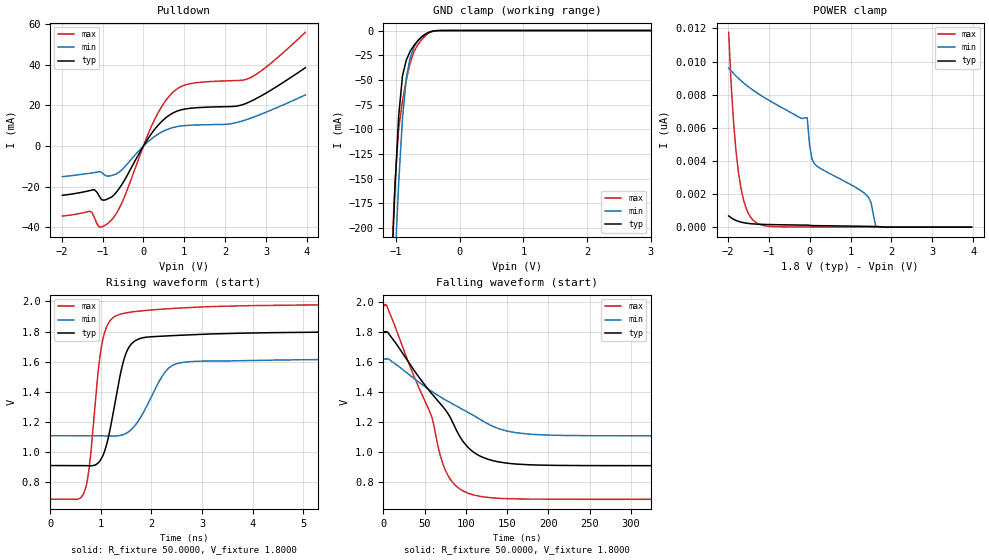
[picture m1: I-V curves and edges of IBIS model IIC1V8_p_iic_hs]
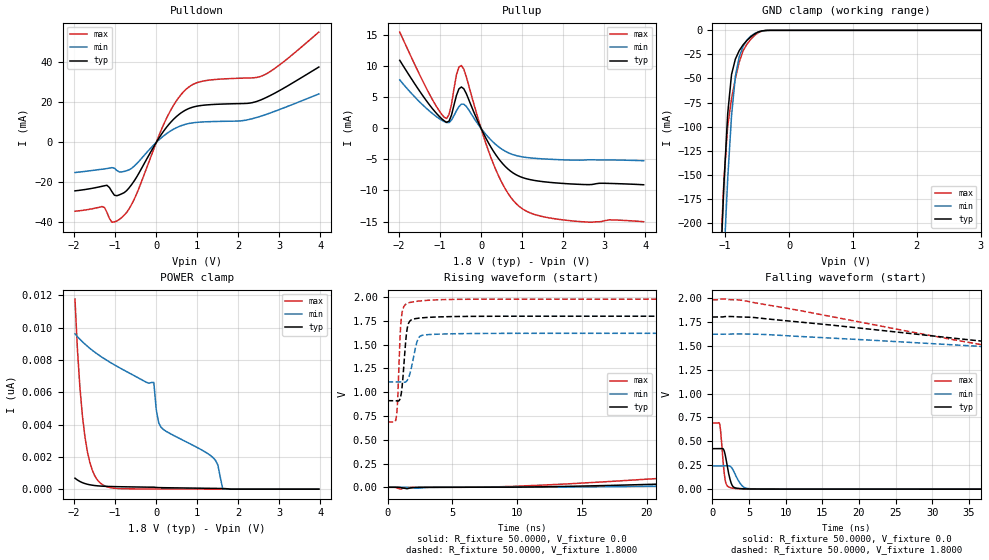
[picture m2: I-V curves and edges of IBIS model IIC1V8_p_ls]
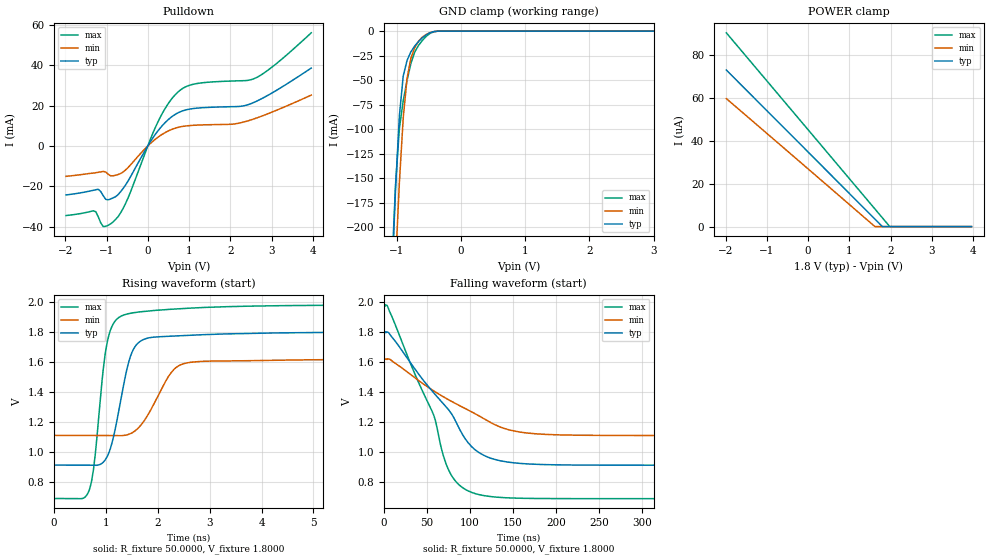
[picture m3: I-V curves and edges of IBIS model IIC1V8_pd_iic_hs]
| IBIS file qfn48_1p8v.ibs generated by Viper version: 2020.12.17
[IBIS Ver]   5.0
[Comment Char]   |_char
[File Name]   qfn48_1p8v.ibs
[File Rev]   1.3
[Date]   Thu Dec 17 17:48:23 2020
[Source]   NXP Viper 2020.12.17
[Notes]
[Disclaimer] IMPORTANT NOTICE
  This information is provided on an AS IS basis and without warranty.
  IN NO EVENT SHALL NXP BE LIABLE FOR INCIDENTAL OR CONSEQUENTIAL
  DAMAGES ARISING FROM USE OF THIS INFORMATION. THIS DISCLAIMER OF
  WARRANTY EXTENDS TO THE USER OF THE INFORMATION, AND TO THEIR CUSTOMERS
  OR USERS OF PRODUCTS  AND IS IN LIEU OF ALL WARRANTIES WHETHER EXPRESS,
  IMPLIED, OR STATUTORY, INCLUDING IMPLIED WARRANTIES OF MERCHANTABILITY
  OR FITNESS FOR PARTICULAR PURPOSE.
  NXP does not represent or warrant that the information furnished
  hereunder is free of infringement of any third party patents,
  copyrights, trade secrets, or other intellectual property rights.
  NXP does not represent or warrant that the information is free of
  defect, or that it meets any particular standard, requirements or need
  of the user of the infomation or their customers.
  NXP reserves the right to change the information in this file
  without notice.
   http://www.nxp.com
[Copyright]   (C) Copyright NXP 2004 - 2020, All Rights Reserved.
|   qfn48
[Component]   qfn48
[Manufacturer]   NXP
[Package]
| variable   typ   min   max
R_pkg   0.17546   0.085233   0.21913
L_pkg   1.979e-9   1.305e-9   2.456e-9
C_pkg   2.005e-13   1.705e-13   3.136e-13
[Pin] signal_name   model_name   R_pin   L_pin   C_pin
1   OPAMP2_INN   NC   0.19686   2.31e-9   1.975e-13
2   P0_1   gpio   0.19885   2.125e-9  1.995e-13
3   P1_0   gpio   0.18462   1.924e-9  1.916e-13
4   P0_11   gpio   0.16868   1.868e-9  1.705e-13
5   VDDIO_1   POWER   NA   NA   NA
6   VDDA   POWER   NA   NA   NA
7   VREF_OUT   NC   0.085233  1.305e-9  2.26e-13
8   VREFP   NC   0.088717  1.309e-9  2.417e-13
9   VREFN   GND   NA   NA   NA
10   P0_16   gpio   0.17435   1.987e-9  1.764e-13
11   P0_10   gpio   0.18496   2.194e-9  1.962e-13
12   P0_15   gpio   0.20527   2.456e-9  2.081e-13
13   P0_8   gpio   0.19119   2.293e-9  1.955e-13
14   OPAMP0_INN   NC   0.1741   2.073e-9  2.101e-13
15   P0_27   gpio   0.16311   1.909e-9  1.814e-13
16   OPAMP1_INN   NC   0.16129   1.801e-9  1.909e-13
17   RESETN   gpio   0.16527   1.717e-9  1.895e-13
18   VDD_CORE   POWER   NA   NA   NA
19   P0_17   gpio   0.16074   1.801e-9  1.861e-13
20   P0_7   gpio   0.1631   1.762e-9  1.925e-13
21   VDDIO_1   POWER   NA   NA   NA
22   VSS_MAIN   GND   NA   NA   NA
23   LX   NC   0.10755   1.361e-9  3.136e-13
24   VDD_MAIN_PWR   NC   NA   NA   NA
25   VBAT   NC   0.21039   2.199e-9  2.126e-13
26   P0_0   gpio   0.19752   2.015e-9  2.122e-13
27   P0_9   gpio   0.17432   1.951e-9  1.886e-13
28   P0_18   gpio   0.16396   1.852e-9  1.719e-13
29   P1_1   gpio   0.1654   1.786e-9  1.75e-13
30   P0_26   gpio   0.16144   1.856e-9  1.764e-13
31   P1_2   gpio   0.16991   1.948e-9  1.848e-13
32   P1_3   gpio   0.18887   2.054e-9  1.928e-13
33   P0_24   gpio   0.17001   1.885e-9  1.791e-13
34   P0_13   iic   0.18016   2.084e-9  1.944e-13
35   P0_14   iic   0.19867   2.298e-9  2.017e-13
36   P0_20   gpio   0.21913   2.324e-9  2.127e-13
37   P0_21   gpio   0.20869   2.216e-9  2.193e-13
38   P0_2   gpio   0.21473   2.265e-9  2.308e-13
39   P0_19   gpio   0.18997   2.14e-9   2.172e-13
40   P0_3   gpio   0.17488   1.926e-9  2.022e-13
41   VDDIO_2   POWER   NA   NA   NA
42   P0_4   gpio   0.16342   1.796e-9  1.814e-13
43   P0_6   gpio   0.16772   1.736e-9  1.992e-13
44   P0_5   gpio   0.16504   1.891e-9  1.879e-13
45   P0_29   gpio   0.16929   1.996e-9  1.98e-13
46   P1_11   gpio   0.18558   2.171e-9  1.964e-13
47   P0_30   gpio   0.20664   2.318e-9  2.205e-13
48   P2_1   gpio   0.1989   2.278e-9  1.972e-13
49   VSS   GND   NA   NA   NA
[Pin Mapping]   pulldown_ref   pullup_ref
1   NC   NC
2   VSS   VDDA
3   VSS   VDDA
4   VSS   VDDA
5   NC   VDDIO_1
6   NC   VDDA
7   NC   NC
8   NC   NC
9   VREFN   NC
10   VSS   VDDA
11   VSS   VDDA
12   VSS   VDDA
13   VSS   VDDA
14   NC   NC
15   VSS   VDDA
16   NC   NC
17   VSS   VDDIO_1
18   NC   VDD_CORE
19   VSS   VDDIO_1
20   VSS   VDDIO_1
21   NC   VDDIO_1
22   VSS_MAIN   NC
23   NC   NC
24   NC   NC
25   NC   NC
26   VSS   VDDIO_2
27   VSS   VDDIO_2
28   VSS   VDDIO_2
29   VSS   VDDIO_2
30   VSS   VDDIO_2
31   VSS   VDDIO_2
32   VSS   VDDIO_2
33   VSS   VDDIO_2
34   VSS   VDDIO_2
35   VSS   VDDIO_2
36   VSS   VDDIO_2
37   VSS   VDDIO_2
38   VSS   VDDIO_2
39   VSS   VDDIO_2
40   VSS   VDDIO_2
41   NC   VDDIO_2
42   VSS   VDDIO_2
43   VSS   VDDIO_2
44   VSS   VDDIO_2
45   VSS   VDDIO_2
46   VSS   VDDIO_2
47   VSS   VDDIO_2
48   VSS   VDDA
49   VSS   NC
|*   Model Selector   *
[Model Selector] gpio
MFIO1V8_pd_hs   EPUN=1 EPD=1 EHS=1
MFIO1V8_pd_ls   EPUN=1 EPD=1 EHS=0
MFIO1V8_pu_hs   EPUN=0 EPD=0 EHS=1
MFIO1V8_pu_ls   EPUN=0 EPD=0 EHS=0
MFIO1V8_p_hs   EPUN=1 EPD=0 EHS=1
MFIO1V8_p_ls   EPUN=1 EPD=0 EHS=0
MFIO1V8_r_hs   EPUN=0 EPD=1 EHS=1
MFIO1V8_r_ls   EPUN=0 EPD=1 EHS=0
[Model Selector] iic
IIC1V8_pd_hs   EGP=1 EPUN=1 EPD=1 EHS=1
IIC1V8_pd_ls   EGP=1 EPUN=1 EPD=1 EHS=0
IIC1V8_p_hs   EGP=1 EPUN=1 EPD=0 EHS=1
IIC1V8_p_ls   EGP=1 EPUN=1 EPD=0 EHS=0
IIC1V8_pu_hs   EGP=1 EPUN=0 EPD=0 EHS=1
IIC1V8_pu_ls   EGP=1 EPUN=0 EPD=0 EHS=0
IIC1V8_r_hs   EGP=1 EPUN=0 EPD=1 EHS=1
IIC1V8_r_ls   EGP=1 EPUN=0 EPD=1 EHS=0
IIC1V8_pd_iic_hs   EGP=0 ECS=0 EPUN=1 EPD=1
IIC1V8_p_iic_hs   EGP=0 ECS=0 EPUN=1 EPD=0
IIC1V8_pu_iic_hs   EGP=0 ECS=0 EPUN=0 EPD=0
IIC1V8_r_iic_hs   EGP=0 ECS=0 EPUN=0 EPD=1
IIC1V8_pd_iic_pu_hs   EGP=0 ECS=1 EPUN=1 EPD=1 SSEL=1
IIC1V8_p_iic_pu_hs   EGP=0 ECS=1 EPUN=1 EPD=0 SSEL=1
IIC1V8_pu_iic_pu_hs   EGP=0 ECS=1 EPUN=0 EPD=0 SSEL=1
IIC1V8_r_iic_pu_hs   EGP=0 ECS=1 EPUN=0 EPD=1 SSEL=1
| End [Component] qfn48
| Models and submodels in the file (24): IIC1V8_p_hs (I/O), IIC1V8_p_iic_hs (I/O_open_drain), IIC1V8_p_iic_pu_hs (I/O_open_drain), IIC1V8_p_ls (I/O), IIC1V8_pd_hs (I/O), IIC1V8_pd_iic_hs (I/O_open_drain), IIC1V8_pd_iic_pu_hs (I/O_open_drain), IIC1V8_pd_ls (I/O), IIC1V8_pu_hs (I/O), IIC1V8_pu_iic_hs (I/O_open_drain), IIC1V8_pu_iic_pu_hs (I/O_open_drain), IIC1V8_pu_ls (I/O), IIC1V8_r_hs (I/O), IIC1V8_r_iic_hs (I/O_open_drain), IIC1V8_r_iic_pu_hs (I/O_open_drain), IIC1V8_r_ls (I/O), MFIO1V8_p_hs (I/O), MFIO1V8_p_ls (I/O), MFIO1V8_pd_hs (I/O), MFIO1V8_pd_ls (I/O), MFIO1V8_pu_hs (I/O), MFIO1V8_pu_ls (I/O), MFIO1V8_r_hs (I/O), MFIO1V8_r_ls (I/O)
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[Model] IIC1V8_p_iic_hs
|   Model IIC1V8_p_iic_hs
| This model was characterised for following simulation conditions:
| External (pad) voltage:
|   - Typ: 1.8V,   - Min: 1.62V,   - Max: 1.98V
| Library cells for typ/min/max conditions are connected as defined below:
|  IO - External Pad
|  A - Core Input
|  EN - Output Buffer Enable
|  BOOST - vdde
|  ECS - gnd
|  EGP - gnd
|  ENZI - vdd
|  EPD - gnd
|  EPUN - vdd
|  ZI - NC
|  ZIF - NC
|  gnd - gnd
|  gnde - gnde
|  vdd - vdd
|  vdde - vdde
| All other pins connected to ground
Model_type I/O_open_drain
Polarity   Non-Inverting
Enable   Active-Low
Vinl =   0.5400V
Vinh =   1.2600V
Vmeas =  0.9000V
Cref =   0.0F
Rref =   1000.000
Vref =   1.8000V
C_comp   3.6454pF   3.5038pF   3.7808pF
|C_comp_pullup   0.9524pF   0.9269pF   0.9624pF
|C_comp_pulldown   2.3410pF   2.4924pF   2.1971pF
[Model Spec]
| variable   typ   min   max
Vinh   0.5400V   0.4860V   0.5940V
Vinl   1.2600V   1.1340V   1.3860V
Vmeas   0.9000V   0.8100V   0.9900V
Vref   1.8000V   1.6200V   1.9800V
Cref   0.0F   0.0F   0.0F
Rref   1.0000k   1.0000k   1.0000k
[Temperature Range]   25.0000   0.1250k   -40.0000
[Voltage Range]   1.8000V   1.6200V   1.9800V
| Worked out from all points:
|   slope of the pulldown table from 0 to 0.27 V, typ, clamps not added: 33.4 ohm
|   GND clamp passes 1 mA (typ) near -0.44 V on its own axis
|   rising waveform, R_fixture 50.0000, V_fixture 1.8000: 20-80 % time 321ps typ, 491ps min, 237ps max; typ from 0.911 V to 1.8 V
|   falling waveform, R_fixture 50.0000, V_fixture 1.8000: 20-80 % time 66.9ns typ, 88.7ns min, 48.9ns max; typ from 1.8 V to 0.911 V
[Pulldown]
|Voltage   I(typ)   I(min)   I(max)
-1.98V    -24.22mA   -15.04mA   -34.42mA
-1.32V    -21.94mA   -13.4mA    -32.06mA
-1.2V     -21.45mA   -13.05mA   -35.06mA
-1.08V    -24.63mA   -12.6mA    -39.9mA
-900mV    -26.23mA   -14.78mA   -38.53mA
-540mV    -19.33mA   -11.9mA    -28.53mA
300mV     8.856mA    5.096mA    14.12mA
720mV     16.26mA    9.117mA    26.48mA
1.14V     18.6mA     10.26mA    30.69mA
2.1V      19.45mA    10.9mA     32.16mA
2.58V     21.61mA    13.44mA    33.34mA
3.96V     38.56mA    25.19mA    55.99mA
[GND_clamp]
|Voltage   I(typ)   I(min)   I(max)
-1.98V    -2.104A    -2.075A    -2.136A
-1.08V    -259.3mA   -333mA     -246.9mA
-1.02V    -161.8mA   -238.7mA   -157.1mA
-960mV    -86.74mA   -154.7mA   -99.46mA
-900mV    -45.95mA   -88.82mA   -71.05mA
-840mV    -29.9mA    -47.99mA   -50.25mA
-780mV    -21.15mA   -27.64mA   -32.98mA
-720mV    -15.16mA   -16.87mA   -21.26mA
-660mV    -10.56mA   -10.24mA   -14.56mA
-540mV    -3.788mA   -3.398mA   -5.292mA
-300mV    -15.94uA   -36uA      -16.34uA
3.96V     0A         0A         0A
[POWER_clamp]
|Voltage   I(typ)   I(min)   I(max)
-1.98V    679.6pA    9.61nA     11.76nA
-1.86V    475.2pA    9.277nA    6.313nA
-1.74V    349.2pA    8.982nA    3.292nA
-1.56V    245.6pA    8.597nA    1.186nA
-1.32V    186pA      8.161nA    293.2pA
-60mV     124.8pA    6.606nA    14.31pA
0V        105.5pA    4.916nA    11.81pA
120mV     93.21pA    3.82nA     10.91pA
1.38V     50pA       1.96nA     2.877pA
1.5V      45.28pA    1.501nA    2.149pA
1.62V     39.18pA    0A         1.42pA
3.96V     0A         0A         0A
[Ramp]
| variable   typ   min   max
dV/dt_r  0.5334/0.3209n   0.3066/0.4909n   0.7753/0.2369n
dV/dt_f  0.5334/66.9323n   0.3066/88.7325n   0.7753/48.9497n
R_load = 50.0000
[Rising Waveform]
R_fixture= 50.0000
V_fixture= 1.8000
V_fixture_min= 1.6200
V_fixture_max= 1.9800
|time   V(typ)   V(min)   V(max)
0s        911mV      1.109V     687.8mV
683.3ps   910.2mV    1.109V     745.5mV
780.5ps   909.1mV    1.109V     927.7mV
1.017ns   961.1mV    1.108V     1.71V
1.277ns   1.32V      1.107V     1.9V
1.506ns   1.663V     1.126V     1.925V
1.797ns   1.757V     1.237V     1.938V
2.547ns   1.776V     1.591V     1.956V
6.124ns   1.798V     1.616V     1.979V
1us       1.8V       1.62V      1.98V
[Falling Waveform]
R_fixture= 50.0000
V_fixture= 1.8000
V_fixture_min= 1.6200
V_fixture_max= 1.9800
|time   V(typ)   V(min)   V(max)
0s        1.8V       1.62V      1.98V
4.033ns   1.8V       1.621V     1.975V
57.1ns    1.4V       1.41V      1.258V
68.97ns   1.323V     1.369V     978.6mV
76.93ns   1.269V     1.343V     860.5mV
95.01ns   1.085V     1.288V     749mV
110.3ns   997.3mV    1.242V     715.6mV
148.2ns   929.5mV    1.144V     692.6mV
208ns     913.4mV    1.113V     688.4mV
1us       911.1mV    1.109V     687.9mV
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[Model] IIC1V8_p_ls
|   Model IIC1V8_p_ls
| This model was characterised for following simulation conditions:
| External (pad) voltage:
|   - Typ: 1.8V,   - Min: 1.62V,   - Max: 1.98V
| Library cells for typ/min/max conditions are connected as defined below:
|  IO - External Pad
|  A - Core Input
|  EN - Output Buffer Enable
|  BOOST - vdde
|  EGP - vdd
|  EHS - gnd
|  ENZI - vdd
|  EPD - gnd
|  EPUN - vdd
|  ZI - NC
|  ZIF - NC
|  gnd - gnd
|  gnde - gnde
|  vdd - vdd
|  vdde - vdde
| All other pins connected to ground
Model_type I/O
Polarity   Non-Inverting
Enable   Active-Low
Vinl =   0.5400V
Vinh =   1.2600V
Vmeas =  0.9000V
Cref =   0.0F
Rref =   1.0000k
Vref =   0.0V
C_comp   3.6452pF   3.5037pF   3.7805pF
|C_comp_pullup   0.9521pF   0.9262pF   0.9623pF
|C_comp_pulldown   2.3411pF   2.4927pF   2.1971pF
[Model Spec]
| variable   typ   min   max
Vinh   0.5400V   0.4860V   0.5940V
Vinl   1.2600V   1.1340V   1.3860V
Vmeas   0.9000V   0.8100V   0.9900V
[Temperature Range]   25.0000   0.1250k   -40.0000
[Voltage Range]   1.8000V   1.6200V   1.9800V
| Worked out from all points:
|   slope of the pulldown table from 0 to 0.27 V, typ, clamps not added: 33.4 ohm
|   slope of the pullup table from 0 to 0.27 V, typ, clamps not added: 80.7 ohm
|   GND clamp passes 1 mA (typ) near -0.44 V on its own axis
|   rising waveform, R_fixture 50.0000, V_fixture 0.0: 20-80 % time 70.1ns typ, 82ns min, 57.1ns max; typ from 0 V to 0.423 V
|   rising waveform, R_fixture 50.0000, V_fixture 1.8000: 20-80 % time 319ps typ, 487ps min, 235ps max; typ from 0.911 V to 1.8 V
|   falling waveform, R_fixture 50.0000, V_fixture 0.0: 20-80 % time 672ps typ, 1.04ns min, 474ps max; typ from 0.423 V to 0 V
|   falling waveform, R_fixture 50.0000, V_fixture 1.8000: 20-80 % time 66.9ns typ, 88.7ns min, 49ns max; typ from 1.8 V to 0.911 V
[Pulldown]
|Voltage   I(typ)   I(min)   I(max)
-1.98V    -24.22mA   -15.04mA   -34.42mA
-1.32V    -21.94mA   -13.4mA    -32.06mA
-1.2V     -21.45mA   -13.05mA   -35.06mA
-1.08V    -24.63mA   -12.6mA    -39.9mA
-900mV    -26.23mA   -14.78mA   -38.53mA
-720mV    -24.07mA   -14.13mA   -34.99mA
-540mV    -19.33mA   -11.9mA    -28.53mA
300mV     8.856mA    5.096mA    14.12mA
720mV     16.26mA    9.117mA    26.48mA
1.14V     18.6mA     10.26mA    30.69mA
2.58V     21.56mA    13.35mA    33.32mA
3.96V     37.73mA    24.28mA    55.2mA
[Pullup]
|Voltage   I(typ)   I(min)   I(max)
-1.98V    10.95mA    7.799mA    15.5mA
-1.32V    4.346mA    3.159mA    6.304mA
-900mV    1.218mA    1.094mA    1.804mA
-780mV    1.156mA    929.2uA    2.224mA
-600mV    5.286mA    2.831mA    8.611mA
-480mV    6.667mA    3.906mA    10.12mA
-420mV    6.372mA    3.889mA    9.539mA
360mV     -4.265mA   -2.608mA   -6.666mA
660mV     -6.57mA    -3.917mA   -10.5mA
960mV     -7.8mA     -4.537mA   -12.74mA
2.04V     -8.889mA   -5.075mA   -14.77mA
3.96V     -9.081mA   -5.209mA   -15.04mA
[GND_clamp]
|Voltage   I(typ)   I(min)   I(max)
-1.98V    -2.104A    -2.075A    -2.136A
-1.08V    -259.3mA   -333mA     -246.9mA
-1.02V    -161.8mA   -238.7mA   -157.1mA
-960mV    -86.74mA   -154.7mA   -99.46mA
-900mV    -45.95mA   -88.82mA   -71.05mA
-840mV    -29.9mA    -47.99mA   -50.25mA
-780mV    -21.15mA   -27.64mA   -32.98mA
-720mV    -15.16mA   -16.87mA   -21.26mA
-660mV    -10.56mA   -10.24mA   -14.56mA
-540mV    -3.788mA   -3.398mA   -5.292mA
-300mV    -15.94uA   -36uA      -16.34uA
3.96V     0A         0A         0A
[POWER_clamp]
|Voltage   I(typ)   I(min)   I(max)
-1.98V    679.6pA    9.61nA     11.76nA
-1.86V    475.2pA    9.277nA    6.313nA
-1.74V    349.2pA    8.982nA    3.292nA
-1.56V    245.6pA    8.597nA    1.186nA
-1.32V    186pA      8.161nA    293.2pA
-60mV     124.8pA    6.606nA    14.31pA
0V        105.5pA    4.916nA    11.81pA
120mV     93.21pA    3.82nA     10.91pA
1.38V     50pA       1.96nA     2.877pA
1.5V      45.28pA    1.501nA    2.149pA
1.62V     39.18pA    0A         1.42pA
3.96V     0A         0A         0A
[Ramp]
| variable   typ   min   max
dV/dt_r  0.2539/70.1178n   0.1457/81.9302n   0.4150/57.0489n
dV/dt_f  0.5334/66.9358n   0.3066/88.6649n   0.7753/48.9538n
R_load = 50.0000
[Rising Waveform]
R_fixture= 50.0000
V_fixture= 0.0
V_fixture_min= 0.0
V_fixture_max= 0.0
|time   V(typ)   V(min)   V(max)
0s        602.8pV    52.95nV    41.9pV
1.012ns   -3.31mV    192.5uV    -19.98mV
1.632ns   -11.39mV   -2.738mV   -1.795mV
12.68ns   6.299mV    1.388mV    27.19mV
45.88ns   145.4mV    64.89mV    304.8mV
84.55ns   285.2mV    143.4mV    561.1mV
103.3ns   339.8mV    172mV      629.2mV
134ns     392.1mV    207.9mV    672.5mV
250.9ns   422.4mV    241.3mV    691.3mV
1us       423.2mV    242.8mV    691.7mV
[Rising Waveform]
R_fixture= 50.0000
V_fixture= 1.8000
V_fixture_min= 1.6200
V_fixture_max= 1.9800
|time   V(typ)   V(min)   V(max)
0s        911mV      1.109V     687.8mV
685.2ps   909.5mV    1.109V     745.1mV
787ps     907.1mV    1.109V     945.8mV
1.007ns   951.3mV    1.108V     1.694V
1.269ns   1.304V     1.105V     1.904V
1.479ns   1.639V     1.118V     1.932V
1.768ns   1.755V     1.218V     1.945V
2.476ns   1.78V      1.585V     1.96V
5.596ns   1.797V     1.616V     1.978V
1us       1.8V       1.62V      1.98V
[Falling Waveform]
R_fixture= 50.0000
V_fixture= 0.0
V_fixture_min= 0.0
V_fixture_max= 0.0
|time   V(typ)   V(min)   V(max)
0s        423.2mV    242.8mV    691.7mV
1.011ns   423.2mV    242.8mV    674.4mV
1.154ns   424.5mV    242.8mV    586.3mV
1.621ns   398.5mV    242.8mV    166.3mV
1.942ns   280.1mV    244.4mV    44.84mV
2.413ns   102.2mV    239.4mV    16.8mV
2.833ns   25.91mV    200.2mV    9.661mV
4.004ns   4.701mV    40.3mV     3.498mV
5.055ns   2.01mV     5.162mV    2.038mV
1us       19.02nV    85.51nV    10.92nV
[Falling Waveform]
R_fixture= 50.0000
V_fixture= 1.8000
V_fixture_min= 1.6200
V_fixture_max= 1.9800
|time   V(typ)   V(min)   V(max)
0s        1.8V       1.62V      1.98V
4.079ns   1.8V       1.623V     1.975V
57.22ns   1.399V     1.41V      1.256V
69.33ns   1.321V     1.367V     971.7mV
77.23ns   1.267V     1.342V     857.4mV
95.69ns   1.079V     1.287V     746.9mV
111ns     994.9mV    1.239V     714.6mV
149.1ns   928.8mV    1.143V     692.4mV
207.1ns   913.6mV    1.113V     688.4mV
1us       911.1mV    1.109V     687.9mV
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[Model] IIC1V8_pd_iic_hs
|   Model IIC1V8_pd_iic_hs
| This model was characterised for following simulation conditions:
| External (pad) voltage:
|   - Typ: 1.8V,   - Min: 1.62V,   - Max: 1.98V
| Library cells for typ/min/max conditions are connected as defined below:
|  IO - External Pad
|  A - Core Input
|  EN - Output Buffer Enable
|  BOOST - vdde
|  ECS - gnd
|  EGP - gnd
|  ENZI - vdd
|  EPD - vdd
|  EPUN - vdd
|  ZI - NC
|  ZIF - NC
|  gnd - gnd
|  gnde - gnde
|  vdd - vdd
|  vdde - vdde
| All other pins connected to ground
Model_type I/O_open_drain
Polarity   Non-Inverting
Enable   Active-Low
Vinl =   0.5400V
Vinh =   1.2600V
Vmeas =  0.9000V
Cref =   0.0F
Rref =   1000.000
Vref =   1.8000V
C_comp   3.6138pF   3.4666pF   3.7547pF
|C_comp_pullup   0.9378pF   0.9163pF   0.9441pF
|C_comp_pulldown   2.3253pF   2.4781pF   2.1797pF
[Model Spec]
| variable   typ   min   max
Vinh   0.5400V   0.4860V   0.5940V
Vinl   1.2600V   1.1340V   1.3860V
Vmeas   0.9000V   0.8100V   0.9900V
Vref   1.8000V   1.6200V   1.9800V
Cref   0.0F   0.0F   0.0F
Rref   1.0000k   1.0000k   1.0000k
[Temperature Range]   25.0000   0.1250k   -40.0000
[Voltage Range]   1.8000V   1.6200V   1.9800V
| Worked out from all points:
|   slope of the pulldown table from 0 to 0.27 V, typ, clamps not added: 33.4 ohm
|   GND clamp passes 1 mA (typ) near -0.44 V on its own axis
|   rising waveform, R_fixture 50.0000, V_fixture 1.8000: 20-80 % time 320ps typ, 490ps min, 236ps max; typ from 0.91 V to 1.8 V
|   falling waveform, R_fixture 50.0000, V_fixture 1.8000: 20-80 % time 66.8ns typ, 88.6ns min, 48.9ns max; typ from 1.8 V to 0.91 V
[Pulldown]
|Voltage   I(typ)   I(min)   I(max)
-1.98V    -24.22mA   -15.04mA   -34.42mA
-1.32V    -21.94mA   -13.4mA    -32.06mA
-1.2V     -21.45mA   -13.05mA   -35.06mA
-1.08V    -24.63mA   -12.6mA    -39.9mA
-900mV    -26.23mA   -14.78mA   -38.53mA
-540mV    -19.33mA   -11.9mA    -28.53mA
300mV     8.856mA    5.096mA    14.12mA
720mV     16.26mA    9.117mA    26.48mA
1.14V     18.6mA     10.26mA    30.69mA
2.1V      19.45mA    10.89mA    32.16mA
2.58V     21.61mA    13.43mA    33.34mA
3.96V     38.53mA    25.17mA    55.97mA
[GND_clamp]
|Voltage   I(typ)   I(min)   I(max)
-1.98V    -2.104A    -2.075A    -2.136A
-1.08V    -259.3mA   -333mA     -246.9mA
-1.02V    -161.8mA   -238.7mA   -157.1mA
-960mV    -86.75mA   -154.7mA   -99.47mA
-900mV    -45.96mA   -88.82mA   -71.06mA
-840mV    -29.91mA   -48mA      -50.26mA
-780mV    -21.16mA   -27.65mA   -32.99mA
-720mV    -15.17mA   -16.88mA   -21.27mA
-660mV    -10.57mA   -10.24mA   -14.57mA
-540mV    -3.796mA   -3.405mA   -5.301mA
-300mV    -21.69uA   -40.85uA   -23.15uA
3.96V     0A         0A         0A
[POWER_clamp]
|Voltage   I(typ)   I(min)   I(max)
-1.98V    73.06uA    59.72uA    90.42uA
1.62V     3.484uA    0A         8.225uA
1.8V      0A         0A         4.113uA
1.98V     0A         0A         0A
3.96V     0A         0A         0A
[Ramp]
| variable   typ   min   max
dV/dt_r  0.5328/0.3204n   0.3064/0.4905n   0.7742/0.2363n
dV/dt_f  0.5327/66.8167n   0.3063/88.5485n   0.7742/48.8803n
R_load = 50.0000
[Rising Waveform]
R_fixture= 50.0000
V_fixture= 1.8000
V_fixture_min= 1.6200
V_fixture_max= 1.9800
|time   V(typ)   V(min)   V(max)
0s        910.3mV    1.108V     687.5mV
683.8ps   909.5mV    1.108V     745.6mV
781ps     908.4mV    1.108V     928.7mV
1.004ns   952.7mV    1.108V     1.684V
1.256ns   1.281V     1.106V     1.895V
1.48ns    1.64V      1.121V     1.922V
1.782ns   1.754V     1.228V     1.936V
2.499ns   1.774V     1.586V     1.954V
5.711ns   1.796V     1.614V     1.976V
1us       1.798V     1.619V     1.978V
[Falling Waveform]
R_fixture= 50.0000
V_fixture= 1.8000
V_fixture_min= 1.6200
V_fixture_max= 1.9800
|time   V(typ)   V(min)   V(max)
0s        1.798V     1.619V     1.978V
4.099ns   1.798V     1.62V      1.972V
58.16ns   1.391V     1.405V     1.24V
68.8ns    1.323V     1.368V     979.5mV
76.88ns   1.268V     1.342V     859.4mV
94.48ns   1.087V     1.289V     749.9mV
110.4ns   995.3mV    1.24V      714.9mV
145.3ns   930.8mV    1.147V     692.8mV
202.8ns   913.2mV    1.113V     688.1mV
1us       910.4mV    1.108V     687.5mV
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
